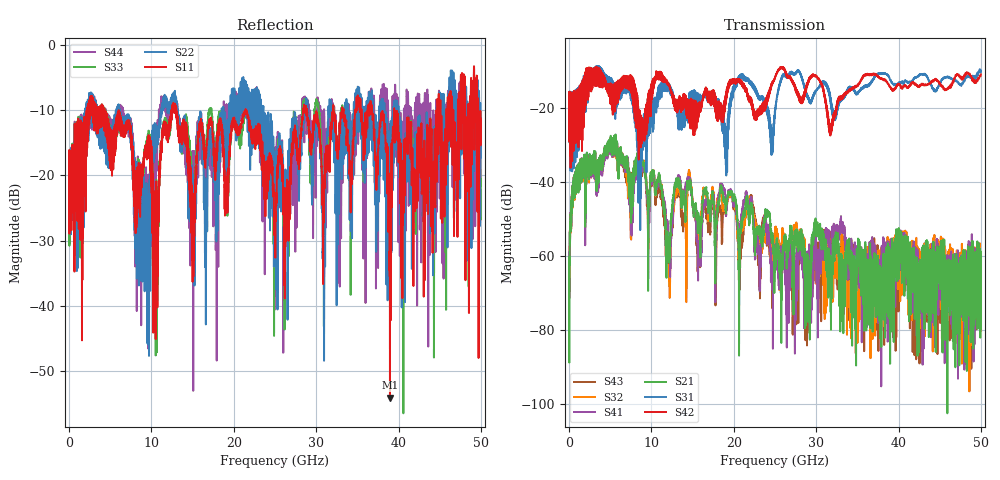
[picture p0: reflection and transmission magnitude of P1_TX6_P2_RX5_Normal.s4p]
!Keysight Technologies,N5225B,MY57041031,A.13.20.10
!Date: Friday, May 31, 2019 11:35:26
!Correction: S11(Full 4 Port(1,2,3,4))
!S12(Full 4 Port(1,2,3,4))
!S13(Full 4 Port(1,2,3,4))
!S14(Full 4 Port(1,2,3,4))
!S21(Full 4 Port(1,2,3,4))
!S22(Full 4 Port(1,2,3,4))
!S23(Full 4 Port(1,2,3,4))
!S24(Full 4 Port(1,2,3,4))
!S31(Full 4 Port(1,2,3,4))
!S32(Full 4 Port(1,2,3,4))
!S33(Full 4 Port(1,2,3,4))
!S34(Full 4 Port(1,2,3,4))
!S41(Full 4 Port(1,2,3,4))
!S42(Full 4 Port(1,2,3,4))
!S43(Full 4 Port(1,2,3,4))
!S44(Full 4 Port(1,2,3,4))
!S4P File: Measurements: <S11,S12,S13,S14>,
!<S21,S22,S23,S24>,
!<S31,S32,S33,S34>,
!<S41,S42,S43,S44>:
# Hz S  dB  R 50.0
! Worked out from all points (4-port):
!   5000 points, 10 MHz to 50 GHz, reference 50 ohm
!   strongest paths, dB at 10 MHz, 12.51 GHz, 25.01 GHz, 37.51 GHz, 50 GHz:
!     S42: -19.5, -16.9, -11.7, -11.6, -11.0
!     S31: -19.3, -15.5, -21.6, -10.8, -9.9
!     S21: -61.3, -47.8, -61.4, -69.2, -67.0
!     S41: -61.2, -51.4, -58.0, -78.2, -69.9
!     S32: -61.6, -51.7, -54.3, -72.1, -66.7
!     S43: -69.4, -53.6, -52.5, -63.8, -63.2
!   lowest |S11| = -54.1 dB at 38.96 GHz (marker M1), VSWR 1.00, Z = 50.1 + j0.177 ohm
!   |S11| at or under -10 dB: 4.286 GHz to 12.47 GHz (8.179 GHz wide, 97.6 % of centre); 13.02 GHz to 21.43 GHz (8.403 GHz wide, 48.8 % of centre); 21.46 GHz to 28.42 GHz (6.96 GHz wide, 27.9 % of centre)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
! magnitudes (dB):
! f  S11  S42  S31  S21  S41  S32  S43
! 10 MHz  -19.5  -19.5  -19.3  -61.3  -61.2  -61.6  -69.4
! 4.96 GHz  -13.2  -15.4  -12.1  -28.9  -29.7  -29.1  -29.6
! 8.62 GHz  -21.0  -26.3  -36.0  -39.0  -39.4  -40.8  -40.7
! 12.08 GHz  -12.6  -13.9  -13.3  -57.3  -54.7  -56.3  -56.9
! 14.59 GHz  -17.1  -20.9  -21.3  -41.0  -39.9  -37.0  -37.8
! 38.96 GHz  -54.1  -14.4  -12.3  -68.7  -61.9  -62.4  -61.7
! 50 GHz  -11.4  -11.0  -9.9  -67.0  -69.9  -66.7  -63.2
